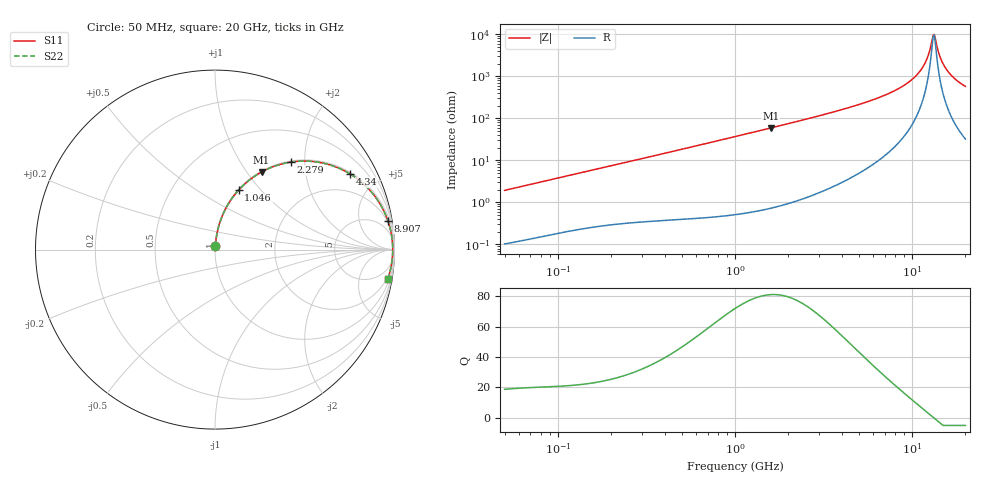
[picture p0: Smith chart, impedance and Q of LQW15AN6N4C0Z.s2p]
!Murata Part Number: LQW15AN6N4C0Z
!These Parameters are Measured in Series Mode Connection
!  o--[Z]--o
!Port1  Port2
!  o-------o
!Freq. Start=50[MHz] Stop=20[GHz], 401[Steps]
# Hz S RI R 50
!Freq.(Hz) S11(Real) S11(Imag) S21(Real) S21(Imag) S12(Real) S12(Imag) S22(Real) S22(Imag)
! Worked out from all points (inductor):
!   401 points, 50 MHz to 20 GHz, reference 50 ohm
!   read as one part in series: L = 6.12 nH near 51.52 MHz
!   highest Q = 81 at 1.591 GHz (marker M1), where L = 5.89 nH
!   self-resonance near 13.15 GHz
!   S11 on the Smith chart (normalised r, x): 50 MHz: 1.00, +0.04; 1.046 GHz: 1.01, +0.77; 2.279 GHz: 1.02, +1.71; 4.34 GHz: 1.07, +3.54; 8.907 GHz: 2, +12; 20 GHz: 2, -11
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5e7  0.0014 0.0193  0.9986 -0.0193  0.9986 -0.0193  0.0014 0.0193
1.364002e8  0.00494 0.0509  0.9951 -0.0509  0.9951 -0.0509  0.00494 0.0509
3.721004e8  0.0218 0.1332  0.9782 -0.1332  0.9782 -0.1332  0.0218 0.1332
1e9  0.1221 0.3205  0.8779 -0.3205  0.8779 -0.3205  0.1221 0.3205
1.045961e9  0.1318 0.3316  0.8682 -0.3316  0.8682 -0.3316  0.1318 0.3316
1.590961e9  0.2598 0.4324  0.7402 -0.4324  0.7402 -0.4324  0.2598 0.4324
2.279204e9  0.4239 0.4877  0.5761 -0.4877  0.5761 -0.4877  0.4239 0.4877
2.728004e9  0.5184 0.4927  0.4816 -0.4927  0.4816 -0.4927  0.5184 0.4927
4.34015e9  0.7539 0.4209  0.2461 -0.4209  0.2461 -0.4209  0.7539 0.4209
7.442007e9  0.9315 0.2331  0.0685 -0.2331  0.0685 -0.2331  0.9315 0.2331
8.907419e9  0.9629 0.1614  0.0371 -0.1614  0.0371 -0.1614  0.9629 0.1614
1.019291e10  0.9784 0.107  0.0216 -0.107  0.0216 -0.107  0.9784 0.107
1.131968e10  0.9859 0.0645  0.0141 -0.0645  0.0141 -0.0645  0.9859 0.0645
1.220001e10  0.989 0.0342  0.011 -0.0342  0.011 -0.0342  0.989 0.0342
1.295331e10  0.9901 0.00991  0.0099 -0.00991  0.0099 -0.00991  0.9901 0.00991
1.314879e10  0.9902 0.00384  0.00981 -0.00384  0.00981 -0.00384  0.9902 0.00384
1.334722e10  0.9902 -0.00223  0.0098 0.00223  0.0098 0.00223  0.9902 -0.00223
1.354865e10  0.9901 -0.00831  0.00986 0.00831  0.00986 0.00831  0.9901 -0.00831
1.460232e10  0.9887 -0.0387  0.0113 0.0387  0.0113 0.0387  0.9887 -0.0387
1.550395e10  0.9862 -0.063  0.0138 0.063  0.0138 0.063  0.9862 -0.063
1.747767e10  0.9776 -0.1115  0.0224 0.1115  0.0224 0.1115  0.9776 -0.1115
2e10  0.9617 -0.166  0.0383 0.166  0.0383 0.166  0.9617 -0.166
